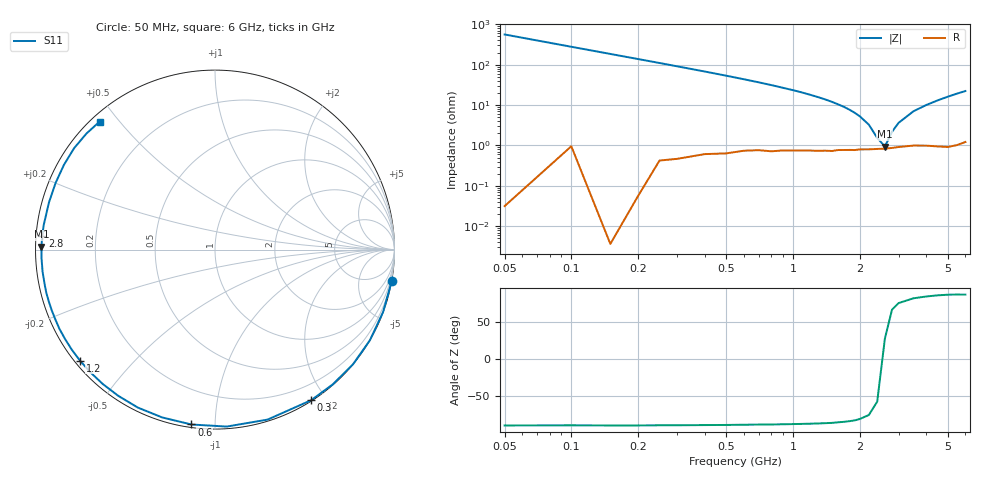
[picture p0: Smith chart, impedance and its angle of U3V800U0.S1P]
! SIEMENS Discrete & RF Semiconductors
! BBY53-02W
! Si Tuning Diode in SCD-80
! VR = 0.8 V
! S-Parameters:  September  1997
# GHz  S  MA  R  50
!  f  S11
! GHz  MAG  ANG
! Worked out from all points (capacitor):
!   34 points, 50 MHz to 6 GHz, reference 50 ohm
!   read as one part to ground: C = 5.72 pF near 50 MHz
!   lowest |Z| = 943 mohm at 2.6 GHz (marker M1)
!   series resonance near 2.55 GHz, so ESL is about 680 pH
!   S11 on the Smith chart (normalised r, x): 50 MHz: 0, -11; 300 MHz: 0.01, -1.83; 600 MHz: 0.01, -0.87; 1.2 GHz: 0.01, -0.36; 2.8 GHz: 0.02, +0.04; 6 GHz: 0.02, +0.45
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0.05  1 -10.2
0.1  0.9988 -20.4
0.15  1 -30.3
0.2  0.9997 -39.8
0.25  0.9971 -48.8
0.3  0.9957 -57.4
0.4  0.9914 -72.8
0.5  0.9881 -86.2
0.6  0.9833 -97.7
0.7  0.9803 -107.5
0.8  0.9795 -116.0
0.9  0.9768 -123.5
1  0.9756 -129.8
1.1  0.9745 -135.4
1.2  0.9738 -140.6
1.4  0.9726 -149.2
1.6  0.9708 -156.5
1.9  0.9701 -165.4
2.2  0.9685 -172.7
2.4  0.9677 -177.0
2.6  0.9671 179.0
2.8  0.9659 175.4
3.5  0.9617 164.1
4  0.9626 157.3
4.5  0.9651 150.7
5  0.9673 144.2
5.5  0.9649 137.9
6  0.96 132.0
